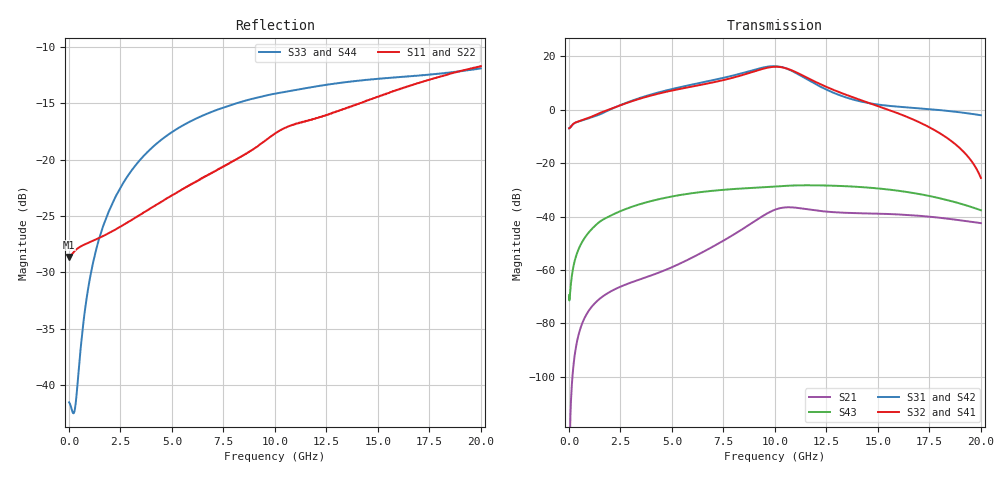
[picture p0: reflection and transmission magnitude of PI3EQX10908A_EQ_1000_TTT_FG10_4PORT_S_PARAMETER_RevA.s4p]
! NPort=4 DATA=2000 NOISE=0 GROUPDELAY=0 COMPLEX_DATAFORMAT=POLAR
! NumOfBlock=1 NumOfParam=0
! .MODEL Smodel S TSTONEFILE=PI3EQX10908A_EQ_1000_TTT_FG10_4PORT_S_PARAMETER_RevA.s4p TYPE=S
!  -- The above .MODEL line can be used for the S element in the netlist.
! The s parameter is extracted from the linear redriver, it is not bi-directional; only s(4,1)s(4,2) and s(3,1)s(3,2)
! should be the insertion loss
!Port definition:
!Port1 = input+
!Port2 = input-
!Port3 = output+
!Port4 = output-
# Hz S MA R  50
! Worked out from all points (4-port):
!   2000 points, 10 MHz to 20 GHz, reference 50 ohm
!   strongest paths, dB at 10 MHz, 5.01 GHz, 10.01 GHz, 15.01 GHz, 20 GHz:
!     S32: -6.9, 7.2, 16.1, 1.4, -25.5
!     S41: -6.9, 7.2, 16.1, 1.4, -25.4
!     S31: -6.9, 7.8, 16.3, 2.0, -2.0
!     S42: -6.9, 7.8, 16.3, 2.0, -2.0
!     S43: -69.4, -32.4, -28.7, -29.5, -37.6
!     S21: -127.2, -58.9, -37.4, -38.9, -42.4
!   lowest |S11| = -28.6 dB at 10 MHz (marker M1), VSWR 1.08, Z = 46.4 - j0.024 ohm
!   |S11| at or under -10 dB: start of sweep to end of sweep
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1e7  0.03701 -179.6  4.34e-07 14.5  0 0.0  0 0.0
     4.34e-07 14.5  0.03701 -179.6  0 0.0  0 0.0
     0.4507 1.0  0.4507 -179.0  0.008374 26.0  0.00034 -27.1
     0.4507 -179.0  0.4507 1.0  0.00034 -27.1  0.008374 26.0
7.11e9  0.08898 -118.9  0.002911 132.8  5.629e-07 59.8  2.735e-07 134.4
        0.002911 132.9  0.08901 -118.9  2.736e-07 134.4  5.63e-07 59.8
        3.669 -53.8  3.332 119.6  0.1652 8.8  0.03082 12.4
        3.333 119.6  3.669 -53.8  0.03082 12.4  0.1652 8.8
9.32e9  0.1176 -111.3  0.009753 112.0  2.991e-06 15.5  1.859e-06 116.8
        0.009759 112.0  0.1176 -111.3  1.86e-06 116.8  2.992e-06 15.4
        6.052 -112.0  5.714 62.4  0.1903 -8.1  0.03518 -10.0
        5.715 62.4  6.053 -112.0  0.03518 -10.0  0.1903 -8.1
1.041e10  0.1372 -111.9  0.01476 74.5  4.587e-06 -18.6  4.898e-06 81.8
          0.01476 74.5  0.1373 -111.9  4.901e-06 81.8  4.588e-06 -18.6
          6.188 -163.4  6.175 10.0  0.1992 -15.3  0.03748 -21.1
          6.175 10.0  6.189 -163.4  0.03748 -21.1  0.1992 -15.3
1.145e10  0.1475 -113.3  0.01394 43.1  5.107e-06 -28.0  7.934e-06 45.1
          0.01394 43.2  0.1476 -113.2  7.939e-06 45.1  5.105e-06 -28.1
          3.935 156.6  4.195 -33.7  0.207 -21.2  0.0386 -33.8
          4.195 -33.7  3.934 156.6  0.0386 -33.8  0.207 -21.2
1.361e10  0.1715 -111.7  0.01173 14.9  1.363e-05 -36.9  1.663e-05 -4.6
          0.01171 15.0  0.1716 -111.7  1.664e-05 -4.6  1.363e-05 -36.9
          1.631 128.0  1.816 -81.0  0.2216 -32.5  0.03684 -60.1
          1.815 -81.0  1.631 128.1  0.03684 -60.1  0.2216 -32.5
2e10  0.2598 -114.6  0.007555 -41.1  8.974e-05 -147.8  7.212e-05 -138.3
      0.007547 -40.7  0.2599 -114.6  7.214e-05 -138.3  8.971e-05 -147.8
      0.7914 56.2  0.05295 171.3  0.2539 -52.2  0.01317 -136.7
      0.05366 172.5  0.7927 56.1  0.01317 -136.7  0.2539 -52.2
